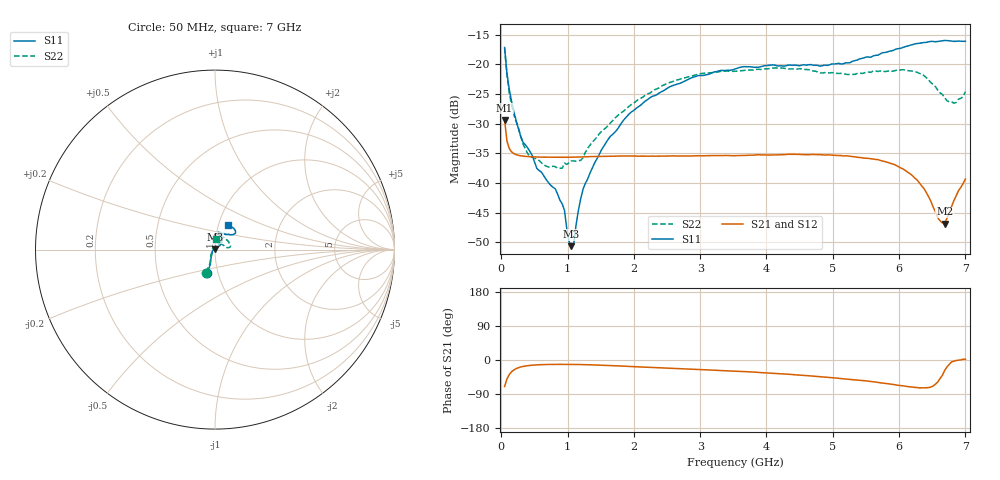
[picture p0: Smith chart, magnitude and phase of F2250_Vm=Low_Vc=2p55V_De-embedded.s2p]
! Integrated Device Technology
! Corporate Headquarters
! 6024 Silver Creek Valley Road
! San Jose, CA 95138  USA
! Phone:  1-408-284-8200
! Toll Free:  1-800-223-1366
! Webpage:  http://www.idt.com/
! Timing and RF Division
! 515 Groton Road, Suite 102
! Westford, MA 01886-6024
! Device:  F2250
! Description: Voltage Variable RF Attenuator
! Frequency:  50.0 -  6000.00 MHz
! Package:  3x3 mm Thin QFN Plastic Package: 16 pin
! Ports:  2 RF, 3 DC
!  Pin  1  = GND
!  Pin  2  = NC
!  Pin  3  = RF1  = Port 1
!  Pin  4  = NC
!  Pin  5  = GND
!  Pin  6  = GND
!  Pin  7  = GND
!  Pin  8  = GND
!  Pin  9  = NC
!  Pin 10  = RF2  = Port 2
!  Pin 11  = NC
!  Pin 12  = GND
!  Pin 13  = GND
!  Pin 14  = VCNTRL
!  Pin 15  = VDD
!  Pin 16  = VMODE
! Vcntrl:  2.550 Volts
! Vmode:  +0.000 Volts
! Vdd:  +3.30  Volts
! Current:  1.174 mA
! Data:  The device was measured on a the F2250 evaluation board which has
!  individual transmission lines to the RF pins.  Data was collected
!  using a calibrated network analyzer.  The evaluation board was
!  de-embedded using a TRL calibration technique.
!  The reference plane is the edge of the package pin.
! Misc:  SN 10
!  Action Tracker AT0258
! Date Measured:  2014-11-26
! Date:  2015-10-15  MJV
! Note:
!  Integrated Device Technology supplies this data as a sample of measured
!  data at the package pin for this product.  Your particular data for this
!  product may vary.
!  Data was taken at 25 degrees C.
!  Integrated Device Technology reserves the right to change this data at anytime.
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# GHz S dB R 50
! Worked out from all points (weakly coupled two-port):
!   201 points, 50 MHz to 7 GHz, reference 50 ohm
!   highest |S21| = -29.41 dB at 50 MHz (marker M1); lowest = -46.9 dB at 6.687 GHz (marker M2)
!   lowest |S11| = -50.7 dB at 1.058 GHz (marker M3), VSWR 1.01, Z = 49.8 + j0.244 ohm
!   |S11| at or under -10 dB: start of sweep to end of sweep
!   |S22| runs from -37.5 to -17.3 dB; largest |S21 - S12| = 5.8e-05
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0.05  -17.18 -108.6  -29.41 -69.8  -29.41 -69.8  -17.28 -111.0
0.08475  -21.44 -107.5  -32.92 -50.4  -32.92 -50.4  -21.75 -110.2
0.15425  -26.23 -116.6  -34.76 -31.1  -34.75 -31.1  -26.82 -122.4
0.29325  -32.20 -127.7  -35.43 -18.5  -35.43 -18.5  -32.09 -137.6
0.3975  -34.09 -141.8  -35.56 -15.0  -35.56 -15.0  -35.04 -160.6
0.91875  -43.53 158.0  -35.69 -11.5  -35.68 -11.5  -37.52 133.4
0.9535  -44.65 170.2  -35.68 -11.5  -35.68 -11.5  -36.66 131.3
1.023  -49.92 144.3  -35.67 -11.6  -35.67 -11.6  -36.61 115.9
1.05775  -50.66 123.5  -35.67 -11.6  -35.67 -11.6  -36.30 110.8
1.0925  -50.31 89.1  -35.66 -11.7  -35.66 -11.7  -36.29 106.3
1.162  -44.70 57.0  -35.64 -11.9  -35.64 -11.9  -36.24 95.6
1.2315  -41.14 44.2  -35.61 -12.1  -35.61 -12.1  -35.78 85.9
1.6485  -32.11 42.0  -35.52 -14.6  -35.52 -14.6  -29.87 64.6
1.9265  -28.39 41.3  -35.47 -16.9  -35.46 -16.9  -27.09 56.8
2.37825  -24.88 47.3  -35.48 -20.3  -35.48 -20.3  -23.99 56.8
3.525  -20.80 72.5  -35.41 -29.5  -35.40 -29.6  -21.19 74.8
4.7065  -20.17 72.3  -35.20 -42.5  -35.21 -42.6  -21.14 72.3
5.85325  -17.81 40.5  -36.63 -63.2  -36.64 -63.3  -21.13 23.0
6.27025  -16.50 40.1  -39.49 -72.6  -39.50 -72.6  -21.36 9.6
6.68725  -15.99 48.8  -46.86 -27.6  -46.82 -27.4  -25.65 28.5
6.861  -16.13 55.1  -42.18 -1.3  -42.13 -1.3  -26.46 57.9
7  -16.12 63.2  -39.35 1.9  -39.30 1.8  -24.62 83.1
